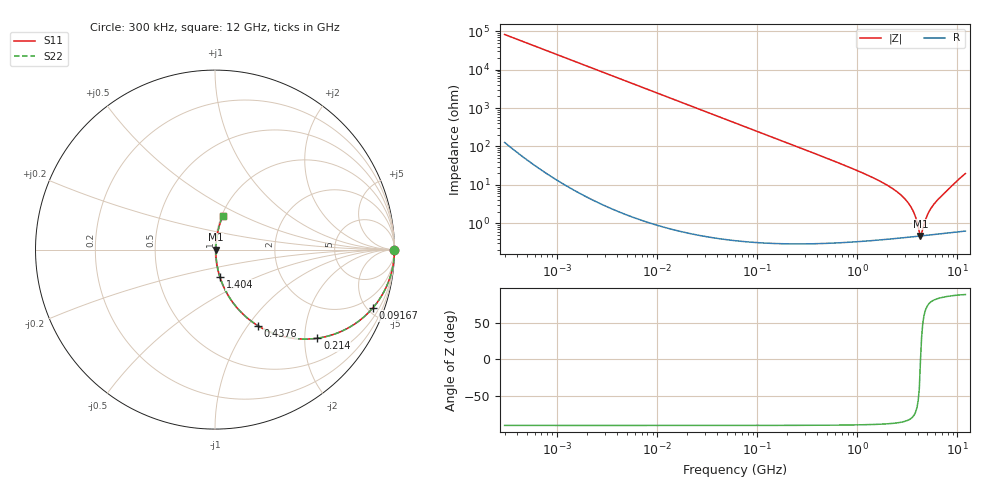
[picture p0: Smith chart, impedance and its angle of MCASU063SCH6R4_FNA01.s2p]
! MCASU063SCH6R4_FNA01  S-PARAMETER MODEL  ( General Type )
! Model Generated by TAIYO YUDEN Corporation (http://www.ty-top.com)
! Version 1.0
! TAIYO YUDEN Control No. 130801
! Copyright(c) 2013 TAIYO YUDEN CO.,LTD. All Rights Reserved.
! Product Description (link to TY-COMPAS)
! https://ds.yuden.co.jp/TYCOMPAS/or/detail?pn=MCASU063SCH6R4DFNA01&u=M
! Products Name : Multilayer Ceramic Capacitors
! Characteristics :
!  Capacitance : 6.4 pF , Rated Voltage : 50V , TCC : CH / C0H
!  Case Size : 0.6 x 0.3 / 0.024 x 0.012 [mm/inch] , Thickness : 0.3 / 0.012 [mm/inch]
!  (Conditions: Temperature = 25 degC , DC Bias Current/Voltage = 0A / 0V)
! External Node Assignments :
!  1  o---| |---o  2
! GND o---------o GND
! Frequency Range : 0.3MHz  -  12000MHz  [ 401 STEP ]
# MHz S RI R 50
! Freq[MHz].  S11 Real  S11 Imag  S21 Real  S21 Imag  S12 Real  S12 Imag  S22 Real  S22 Imag
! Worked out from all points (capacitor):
!   401 points, 300 kHz to 12 GHz, reference 50 ohm
!   read as one part in series: C = 6.43 pF near 316.3 kHz
!   lowest |Z| = 466 mohm at 4.271 GHz (marker M1)
!   series resonance near 4.275 GHz, so ESL is about 220 pH
!   S11 on the Smith chart (normalised r, x): 300 kHz: open; 91.67 MHz: 1.01, -5.40; 214 MHz: 1.01, -2.31; 437.6 MHz: 1.01, -1.12; 1.404 GHz: 1.01, -0.31; 12 GHz: 1.01, +0.39
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0.3  1 -0.00121  3.34e-06 0.00121  3.34e-06 0.00121  1 -0.00121
1.769972  0.9999 -0.00715  5.4e-05 0.00715  5.4e-05 0.00715  0.9999 -0.00715
10.44266  0.9982 -0.0421  0.00179 0.0421  0.00179 0.0421  0.9982 -0.0421
27.10171  0.9881 -0.1082  0.0119 0.1082  0.0119 0.1082  0.9881 -0.1082
60  0.9443 -0.229  0.0557 0.229  0.0557 0.229  0.9443 -0.229
91.67136  0.8789 -0.3256  0.1211 0.3256  0.1211 0.3256  0.8789 -0.3256
213.9924  0.5707 -0.4937  0.4293 0.4937  0.4293 0.4937  0.5707 -0.4937
353.9943  0.3259 -0.4666  0.6741 0.4666  0.6741 0.4666  0.3259 -0.4666
437.5599  0.2397 -0.4242  0.7603 0.4242  0.7603 0.4242  0.2397 -0.4242
743.2595  0.0967 -0.2908  0.9033 0.2908  0.9033 0.2908  0.0967 -0.2908
1403.667  0.0275 -0.1526  0.9725 0.1526  0.9725 0.1526  0.0275 -0.1526
2088.533  0.0119 -0.0891  0.9881 0.0891  0.9881 0.0891  0.0119 -0.0891
2722.03  0.00703 -0.0539  0.993 0.0539  0.993 0.0539  0.00703 -0.0539
3276.641  0.0053 -0.0314  0.9947 0.0314  0.9947 0.0314  0.0053 -0.0314
3642.919  0.0048 -0.019  0.9952 0.019  0.9952 0.019  0.0048 -0.019
4050.141  0.00461 -0.00682  0.9954 0.00682  0.9954 0.00682  0.00461 -0.00682
4270.516  0.00463 -0.000117  0.9954 0.000117  0.9954 0.000117  0.00463 -0.000117
4502.883  0.00473 0.00534  0.9953 -0.00534  0.9953 -0.00534  0.00473 0.00534
5140.631  0.00521 0.0182  0.9948 -0.0182  0.9948 -0.0182  0.00521 0.0182
5868.704  0.00606 0.0315  0.9939 -0.0315  0.9939 -0.0315  0.00606 0.0315
9454.42  0.0182 0.1102  0.9818 -0.1102  0.9818 -0.1102  0.0182 0.1102
12000  0.0427 0.1868  0.9573 -0.1868  0.9573 -0.1868  0.0427 0.1868
